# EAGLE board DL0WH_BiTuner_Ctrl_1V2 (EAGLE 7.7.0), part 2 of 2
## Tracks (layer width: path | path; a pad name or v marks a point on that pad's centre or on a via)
+3V3  (via drill 0.3)
  Top 0.152: R0913.2 10.48,30.48 13.02,33.02 | 19.21,26.83 18.72,27.32 R0971.1 15.24,27.94 v15.56,28.26 | 8.27,27.61 v8.26,27.62
  Top 0.254: U0601.3 28.18,45.95 27.94,45.72 | U0701.3 44.69,45.95 44.45,45.72 | U0801.3 61.2,45.95 60.96,45.72 | C0601.2 27.78,45.09 27.73,45.14 27.04,45.14 26.04,44.13 v26.04,42.55 | C0701.2 44.03,45.3 42.55,43.81 v42.55,42.55 | C0801.2 60.54,45.3 59.05,43.81 v59.05,42.55 | v13.97,16.51 13.64,16.84 U0961.5 17.62,21.74 17.62,23.34 16.67,24.29
  Top 0.305: C1311.1 28.26,37.47 27.62,37.47 v26.67,36.83 | L1311.1 L1311.3 v26.67,36.83 | U1301.5 13.29,41.23 v13.34,41.27 | 27.94,45.72 C0601.2 | 44.45,45.72 C0701.2 | 60.96,45.72 C0801.2 | X0222.1 71.28,30.96 71.44,30.8 R0511.2 R0512.2 | v71.44,19.68 68.26,19.68 v67.94,19.37 | v26.67,36.83 26.67,33.34 26.35,33.02 25.4,33.02 | 25.4,33.02 13.02,33.02 | 24.61,32.23 19.21,26.83 16.67,24.29 16.19,23.81 8.41,23.81 8.26,23.97 8.26,26.67 R0903.2 8.27,27.61 | L0941.2 24.56,32.23 v23.34,32.23 24.61,32.23 | 25.4,33.02 24.61,32.23
  Bottom 0.152: 75.56,4.13 75.56,6.02 | v67.94,19.37 67.94,19.1 SJ0401.1 | C0951.1 15.89,28.59 v15.56,28.26 14.63,27.33 U0951.5 | 22.28,34.12 C0941.1 | U0962.14 13.89,14.61 | 12.08,14.14 C0962.1 | U0962.8 13.98,10.79 15.08,10.79 15.24,10.95 15.24,12.7 | 15.24,12.7 15.24,14.45 15.06,14.62 U0962.14 | U0962.11 13.94,12.7 15.24,12.7 | U0962.14 13.97,14.69
  Bottom 0.254: U0921.8 7.9,27.98 v8.26,27.62 | 13.89,14.61 12.54,14.61 12.08,14.14 | 13.97,14.69 v13.97,16.51
  Bottom 0.305: v26.67,36.83 26.67,38.42 R1321.2 R1322.2 26.04,41.27 26.25,41.91 | v13.34,41.27 17.78,41.27 19.05,42.55 v26.04,42.55 26.25,42.33 26.25,41.91 | v59.05,42.55 59.05,41.91 58.74,41.59 58.42,41.59 | 26.25,41.91 26.35,41.81 26.35,41.59 42.55,41.59 | 75.56,4.13 75.88,3.81 79.38,3.81 X0201.1 | 75.56,6.02 R0231.2 74.92,7.29 74.93,9.21 74.93,19.37 74.61,19.68 73.66,19.68 | v71.44,19.68 73.66,19.68 | 58.42,41.59 58.42,31.11 58.58,30.96 X0222.1 73.5,30.96 73.66,30.8 73.66,19.68 | C0921.1 8.56,27.32 v8.26,27.62 | 42.55,41.59 58.42,41.59 | v42.55,42.55 42.55,41.59 | 22.28,34.12 U0941.5 U0941.4 v23.35,32.24 v23.34,32.23
+5V  (via drill 0.3)
  Top 0.152: U1101.16 43.88,11.43 C1101.1 | 11.75,47.62 L1211.1
  Top 0.254: U1301.1 16.24,40.37 v15.88,40.01 15.24,39.37 U1301.8
  Top 0.305: U1201.9 9.26,57.52 8.89,57.15 8.89,52.07 12.04,48.92 L1211.1 v13.34,47.62 | U1301.1 16.24,41.64 v17.14,42.55 | 11.75,47.62 3.81,47.62 1.27,44.45 1.27,14.29 8.26,7.3 | 8.26,7.3 14.29,1.27 47.62,1.27 47.94,1.59 47.94,7.94 46.35,9.53 46.35,11.12 C1101.1 | 8.26,7.3 35.24,34.29 78.74,34.29 82.55,30.48 | U1001.16 85.41,48.9 86.36,49.85 86.36,51.12 C1001.1 86.38,51.44 94.61,51.44 94.93,51.12 94.93,30.8 94.61,30.48 82.55,30.48 | 82.55,30.48 arc60 D1221.C
  Bottom 0.152: 14.82,35.14 15.24,35.56 15.24,39.37 v15.88,40.01
  Bottom 0.305: C1222.1 C1223.1 13,45.73 13.02,45.09 13.34,44.77 15.88,44.77 16.19,44.45 16.19,43.5 C1301.1 16.51,43.18 v17.14,42.55 | C1222.1 C1221.1 13.34,50.5 13.34,51.44 17.14,51.44 19.04,53.33 R1211.2 | C1222.1 13.32,47.64 v13.34,47.62 | R1302.2 14.82,35.14
+12V  (via drill 0.3)
  Top 0.254: U0601.6 30.12,46.08 30.48,45.72 | C0603.1 32.28,45.3 32.07,45.09 30.64,45.09 30.62,45.1 C0602.1 | U0701.6 46.63,46.08 46.99,45.72 | C0703.1 48.79,45.3 48.58,45.09 47.15,45.09 47.13,45.1 C0702.1 | U0801.6 63.15,46.08 63.5,45.72 | C0803.1 65.3,45.3 65.09,45.09 63.66,45.09 63.64,45.1 C0802.1
  Top 0.305: C0602.1 30.48,45.72 v31.43,45.72 | C0702.1 46.99,45.72 v47.94,45.72 | C0802.1 63.5,45.72 v64.45,45.72 | U1201.11 10.5,56.22 v10.16,55.88 | U1201.12 10.47,55.57 v10.16,55.88 | U1201.13 10.5,54.92 10.16,55.26 v10.16,55.88
  Bottom 0.305: 7.62,55.24 C1202.1 | C1204.1 v10.16,55.88 11.43,57.15 11.43,58.42 12.7,59.69 21.59,59.69 22.86,58.42 22.86,46.99 24.13,45.72 v31.43,45.72 v47.94,45.72 v64.45,45.72 70.48,45.72 78.74,53.98 78.74,64.77 | 78.74,64.77 X1602.17 X1602.18 X1602.20 X1602.19 78.74,64.77
  Bottom 0.406: C1204.1 C1203.1 C1202.1 C1201.1 5.73,55.88 X1211.1
-1V5  (via drill 0.3)
  Top 0.152: 36.45,37.88 L0943.1
  Top 0.254: U0961.2 12.7,21.91 13.03,22.24 C0952.1 12.7,22.72 v12.7,23.02
  Top 0.305: C0943.1 36.45,37.88 | v36.2,37.47 36.2,38.05 L0943.1 | v12.7,23.02 v16.67,23.02 | v33.34,30.48 v29.53,26.67
  Bottom 0.254: v12.7,23.02 U0951.2
  Bottom 0.305: C0945.2 R0945.2 33.34,30.97 v33.34,30.48 | C0945.2 32.07,33.5 | C0945.2 33.18,33.5 36.2,36.51 v36.2,37.47 | v29.53,26.67 20.32,26.67 v16.67,23.02
CAT_DTE_CTS
  Top 0.152: X1153.1 33.66,14.61 35.88,14.61 36.2,14.92 U1101.7
  Bottom 0.152: C1153.1 22.01,4.66 X1153.1
CAT_DTE_RTR
  Top 0.152: X1153.2 30.54,16.57 U1101.8
  Bottom 0.152: C1154.1 16.93,4.66 X1153.2
CAT_DTE_RXD
  Top 0.152: U1101.14 41.27,8.26 X1151.1
  Bottom 0.152: C1151.1 44.87,4.66 X1151.1
CAT_DTE_TXD
  Top 0.152: U1101.13 40.01,4.45 X1151.2
  Bottom 0.152: C1152.1 39.79,4.66 X1151.2
CAT_MX_C1N
  Top 0.152: C1102.2 46.04,14.61 41.59,14.61 41.27,14.92 U1101.3
CAT_MX_C1P
  Top 0.152: U1101.1 44.2,16.51 C1102.1
CAT_MX_C2M
  Top 0.152: U1101.5 38.73,18.41 40.01,19.69 C1103.2
CAT_MX_C2P
  Top 0.152: U1101.4 40.01,18.1 41.27,19.68 C1103.1
CAT_MX_VM
  Top 0.152: U1101.6 37.47,18.73 36.51,19.69 C1105.1
CAT_MX_VP
  Top 0.152: U1101.2 42.55,18.41 44.45,20.32 C1104.1
GND  (via drill 0.3)
  Top 0.152: U0601.7 U0601.8 31.43,47.94 v31.75,48.26 32.08,47.94 U0601.9 U0601.10 | U0701.7 U0701.8 47.94,47.94 v48.26,48.26 48.59,47.94 U0701.9 U0701.10 | U0801.7 U0801.8 64.44,47.94 v64.77,48.26 65.09,47.94 U0801.9 U0801.10 65.75,46.7 65.72,46.67 | 32.7,56.2 32.7,56.7 U0601.23 | 30.8,56.2 30.8,56.7 U0601.26 | U0601.25 31.43,56.2 | U0601.24 32.08,56.2 32.07,56.2 | U0801.26 63.8,56.22 63.82,56.2 | U0801.25 64.44,56.2 64.45,56.2 | U0801.24 65.09,56.2 | U0801.23 65.75,56.22 65.72,56.2 | S0212.1 | 57.78,17.94 57.61,18.1 C0311.2 | U0101.31 71.84,14.21 71.75,14.29 70.8,14.29 70.48,14.61 v70.48,16.51 66.99,16.51 v66.04,17.14 | U0101.63 65.34,23.25 v67.31,21.27 | R0441.1 59.05,16.67 | 53.02,3.87 H1721.B3,0 53.02,3.81 | 84.45,51.12 C1001.2 | 64.14,30.8 C0451.2 63.18,30.8 | 57.96,29.21 C0331.+ | C0803.2 65.83,43.6 66.04,43.81 | v14.61,28.26 13.97,27.62 D0971.C 14.42,26.67 17.46,26.67 v17.62,26.51 | v30,37.47 30,36.67 30.16,36.51 | U0961.3 11.73,20.32 | C0952.2 11.76,22.36
  Top 0.254: 14.61,43.18 15.24,42.55 U1301.3 15.24,40.64 14.74,39.82 U1301.7 14.74,36.06 | U1301.10 16.24,35.92 | U0701.10 49.23,46.65 50.16,45.72 50.16,44.45 49.53,43.81 49.11,43.81 C0703.2 | 32.49,43.6 C0603.2 32.6,43.81 33.02,43.81 33.66,44.45 33.66,45.72 32.73,46.65 U0601.10 | U0701.26 47.28,56.22 47.31,56.2 | U0701.23 49.23,56.22 49.21,56.2 | U0701.25 47.94,56.2 | U0701.24 48.59,56.2 48.58,56.2 | X1401.GND 89.88,22.89 v89.85,22.86 | 65.72,43.81 66.04,43.81 66.36,43.81 66.67,44.13 66.67,45.72 65.72,46.67 | 11.73,20.32 X1501.4 | 11.76,22.36 U0961.3
  Top 0.305: U1201.10 9.88,56.87 v9.72,56.77 | U1201.6 17.78,56.22 | 17.78,56.22 18.12,56.22 18.41,56.52 | 18.41,56.52 20.3,56.52 C1205.1 v20.32,57.78 v17.46,60.64 | U1201.7 18.06,56.87 18.41,56.52 | 18.41,56.52 17.78,56.22 | U1201.15 10.44,53.62 v10.16,53.34 | U1201.16 10.53,52.97 v10.16,53.34 | v13.34,43.18 14.61,43.18 v14.61,48.9 14.61,51.44 14.29,51.75 14.29,52.07 | 16.24,35.92 15.88,35.56 15.24,35.56 14.74,36.06 | v17.14,36.83 16.51,36.83 16.51,36.9 U1301.10 | C0601.1 28.1,43.66 28.16,43.6 28.79,43.6 v29.21,43.18 | C0603.2 32.23,43.81 30.96,43.81 30.94,43.8 C0602.2 30.32,43.66 30.27,43.6 29.63,43.6 v29.21,43.18 | v28.57,34.92 C1311.2 28.89,35.88 29.84,35.88 30.16,36.2 30.16,36.51 30.16,40.64 | C0701.1 44.45,43.66 44.51,43.6 45.3,43.6 v45.72,43.18 | v45.72,43.18 46.14,43.6 46.77,43.6 46.83,43.66 C0702.2 47.13,43.8 47.15,43.81 48.58,43.81 48.79,43.6 C0703.2 | C0803.2 65.3,43.6 65.09,43.81 63.66,43.81 63.64,43.8 C0802.2 63.34,43.66 63.28,43.6 62.65,43.6 v62.23,43.18 | C0801.1 61.12,43.66 61.17,43.6 61.81,43.6 v62.23,43.18 | U1201.PAD4 14.29,52.07 | 14.29,52.07 10.48,52.07 10.16,52.39 v10.16,53.34 | v29.21,43.18 29.21,40.96 29.53,40.64 30.16,40.64 | 30.16,40.64 38.89,40.64 | 38.89,40.64 45.72,40.64 | 45.72,40.64 61.91,40.64 62.23,40.96 | 62.23,40.96 v62.23,43.18 | 45.72,40.64 v45.72,43.18 | 30.8,56.2 31.43,56.2 31.75,56.2 | 31.75,56.2 32.07,56.2 32.7,56.2 | 31.75,56.2 U0601.33 | U0701.33 48.26,56.2 | 48.26,56.2 47.94,56.2 47.31,56.2 | 48.26,56.2 48.58,56.2 49.21,56.2 | 63.82,56.2 64.45,56.2 64.77,56.2 | 64.77,56.2 65.09,56.2 65.72,56.2 | v64.77,51.44 U0801.33 64.77,56.2 | S0212.1 65.72,5.08 65.41,5.4 C0213.2 65.34,7.86 65.34,13.27 U0101.18 65.34,16.44 v66.04,17.14 66.36,17.46 66.36,20.32 66.67,20.64 66.99,20.64 67.31,20.95 v67.31,21.27 67.94,21.91 v72.07,21.91 72.42,22.3 U0101.47
  Top 0.305: S0212.1 v68.9,4.45 | R0441.1 58.09,17.77 57.78,17.94 | 59.05,16.67 v59.21,16.67 | 53.02,3.87 49.21,7.62 49.21,11.11 48.9,11.43 v48.58,11.43 C1101.2 | U1101.15 42.55,8.26 v44.77,6.03 | C1105.2 34.61,20.32 34.61,21.27 35.24,21.91 46.04,21.91 46.35,21.59 46.35,21.27 C1104.2 v46.99,20.32 | X1052.1 90.81,47.62 U1001.15 83.82,47.62 83.03,47.94 83.03,50.01 83.66,50.48 84.45,51.12 | 62.23,40.96 62.55,40.64 74.93,40.64 74.93,40.95 C1005.2 74.93,52.39 75.25,52.7 82.55,52.7 82.87,52.39 82.87,51.12 | C1001.2 82.87,51.12 | 82.87,51.12 C1004.2 | 64.14,30.8 v64.77,30.16 65.09,29.84 65.09,27.46 65.34,27.21 U0101.63 | 63.18,30.8 61.59,29.21 60.96,29.21 | 60.96,29.21 57.96,29.21 | C0332.2 60.96,29.21 | v48.58,14.61 57.44,14.61 v58.42,14.27 | C0943.2 38.73,40.48 38.89,40.64
  Bottom 0.152: R1301.1 X1511.3 | C1223.2 C1222.2 | 59.52,15.48 C0412.2 | C0410.2 71.44,21.27 v72.07,21.91 | C0402.2 70.47,16.21 v70.48,16.51 | C0401.2 66.34,17.16 v66.04,17.14 | C0403.2 67.25,21.53 v67.31,21.27 | 59.28,16.6 v59.21,16.67 | R0221.1 v64.77,30.16 | 14.59,31.11 C0951.2 14.59,28.27 v14.61,28.26 | C1152.2 38.1,1.27 | C1151.2 43.18,1.27 | C1154.2 15.24,1.27 | C1153.2 20.32,1.27 | C1051.2 93.88,63.18 94.93,63.18 | C1052.2 94.93,58.42 | C1053.2 93.88,40.32 95.25,40.32 | C0054.2 95.25,35.56 | v17.14,36.83 17.14,34.61 17.62,34.13 C0941.2 | D0942.C v30,37.47 32.07,35.4 32.07,34.78 R0946.1 | U0941.2 28.26,33.18 28.57,33.5 v28.57,34.92 | v10.16,33.02 11.43,34.29 | C0962.2 10.79,13.96 10.79,13.18 | 10.79,13.18 12.7,13.18 12.85,13.32 U0962.12 U0962.13 13.96,13.97 13.97,13.97 | U0962.4 17.96,12.68 17.94,12.7 | 17.94,12.7 17.78,12.86 17.78,14.45 17.94,14.61 19.09,14.61 U0962.1 | 17.94,12.7 15.24,10 11.59,10 11.43,10.16 11.43,11.91 10.79,12.54 10.79,13.18
  Bottom 0.254: U0921.4 4.65,29.96 | C0962.2 9.51,15.24 X1501.3
  Bottom 0.305: C1212.2 20.3,57.8 v20.32,57.78 | v10.16,53.34 C1204.2 C1203.2 C1202.2 C1201.2 | C1301.2 v13.34,43.18 12.38,41.91 X1511.4 | X1211.2 9.72,60.96 | 9.72,60.96 v9.72,56.77 | X1211.2 H1751.B3,0 6.35,71.12 90.81,71.12 H1761.B3,0 94.93,66.99 94.93,63.18 94.93,58.42 94.93,53.66 92.71,51.44 X1052.1 X1052.2 95.25,41.91 95.25,40.32 95.25,35.56 95.25,30.48 91.44,26.67 89.22,26.67 C1403.1 89.2,25.4 C1403.1 | X1501.2 H1711.B3,0 6.35,1.27 15.24,1.27 20.32,1.27 26.99,1.27 X1152.2 X1152.1 36.83,1.27 38.1,1.27 43.18,1.27 50.55,1.27 H1721.B3,0 | X1501.2 X1501.3 X1501.4 11.76,23.19 11.76,23.81 | X1501.5 X1501.2 | X1501.5 3.81,21.91 4.23,22.33 C0901.2 R0901.1 | U0951.3 11.76,23.81 | C0921.2 10.16,24.77 11.11,23.81 11.76,23.81 | X1511.2 3.81,34.71 C0911.2 R0911.1 4.13,32.28 4.13,30.48 4.65,29.96 | X1511.5 X1511.4 | X1511.2 X1511.5 | X1511.4 X1511.3 11.43,34.29 v13.97,31.75 14.45,31.27 14.59,31.11 | C1222.2 C1221.2 v14.62,48.91 v14.61,48.9 | X1211.2 1.27,58.42 1.27,44.45 X1511.5 | 9.72,60.96 17.46,60.96 | 17.46,60.96 21.59,60.96 30.48,52.07 U0601.33 v31.75,48.26 | v17.46,60.64 17.46,60.96 | v48.26,48.26 U0701.33 | v64.77,48.26 v64.77,51.44 | H1731.B3,0 92.71,15.24 v90.17,17.78 90.17,22.54 v89.85,22.86 87,22.86 86.68,23.18 86.68,25.08 87,25.4 87.77,25.4 R1402.1 C1403.1 | v68.9,4.45 71.75,4.45 72.55,5.24 R0232.1 74.92,3.51 75.56,2.86 80.96,2.86 81.28,3.17 X0201.3 X0201.5 82.55,3.17 82.87,2.86 84.77,2.86 85.09,3.17 85.09,3.81 | 59.52,15.48 59.21,15.4 59.04,15.22 C0413.2 58.9,13.81 v58.42,14.27 | X0601.2 X0601.4 85.09,30.48 89.22,26.35 C1403.1 | C0412.2 59.37,15.56 59.37,16.51 59.28,16.6
  Bottom 0.305: v44.77,6.03 50.8,6.03 55.56,1.27 90.17,1.27 H1731.B3,0 | v48.58,11.43 v48.58,14.61 48.58,18.73 v46.99,20.32 | X1501.5 2.54,21.59 2.54,35.56 X1511.2 | 85.09,3.81 X0201.9 | 85.09,3.81 H1731.B3,0
  other vias: 31.75,52.07 48.26,52.07 55.88,20.32 68.58,58.42
  pour Top: 0.32,3.32 0.32,69.71 arc-88 3,72.71 93.2,72.71 arc-98 96.2,69.71 96.2,3.32 arc-88 93.2,0.32 3,0.32 arc-78
  pour Bottom: 0.32,3.32 0.32,69.71 arc-88 3,72.71 93.2,72.71 arc-98 96.2,69.71 96.2,3.32 arc-88 93.2,0.32 3,0.32 arc-78
LM2611_NFB
  Bottom 0.152: R0946.2 C0945.1 R0945.1 U0941.3
LM2611_SW  (via drill 0.3)
  Top 0.305: C0942.1 30.21,33.02 29.23,32.05 | 29.23,32.05 L0941.1 | v27.78,34.13 27.78,33.66 28.1,33.34 28.1,33.18 29.23,32.05
  Bottom 0.305: U0941.1 27.77,34.12 v27.78,34.13
LM53603_BIAS  (via drill 0.3)
  Top 0.152: U1201.5 18.74,55.57 19.05,55.88 v21.59,55.88
  Bottom 0.152: R1211.1 19.7,55.26 20.32,55.88 v21.59,55.88
  Bottom 0.305: R1211.1 C1212.1
LM53603_CBOOT
  Top 0.152: U1201.3 19.39,54.27 20,53.66 20.3,53.34
  Top 0.305: 20.3,53.34 C1211.2
LM53603_SW
  Top 0.152: 18.41,52.97 19.1,52.97 19.68,52.39 20.3,52.07
  Top 0.305: U1201.1 18.41,52.97 18.41,53.34 18.14,53.62 U1201.2 | 20.3,52.07 C1211.1
  Top 0.406: L1211.2 16.54,50.19 18.41,52.07 18.41,52.97
LM53603_VCC
  Top 0.152: U1201.4 19.36,54.92 19.68,55.24 20.3,55.24
  Top 0.305: 20.3,55.24 C1205.2
LM_DA  (via drill 0.3)
  Top 0.305: C0942.2 31.43,35.4 32.54,36.51 v32.54,37.47 L0943.2
  Bottom 0.305: v32.54,37.47 32.54,37.9 D0942.A
MCU_NRST  (via drill 0.3)
  Top 0.152: C0213.1 61.59,7.62 61.28,7.3 S0212.2 | C0213.1 64.14,9.51 64.14,4.13 64.45,3.81 71.12,3.81 74.45,7.14 84.14,7.14 85.09,6.19 X0201.10 | U0101.7 63.28,19.75 63.18,19.84 v64.29,19.84 | C0213.1 64.12,10.46 v64.14,12.06
  Bottom 0.152: v64.14,12.06 64.14,13.34 64.77,13.97 64.77,19.37 v64.29,19.84
MCU_VBAT
  Top 0.152: U0101.1 63.13,22.75 63.18,23.5 63.18,26.99 TP_VBAT.TP C0451.1
MCU_VDD  (via drill 0.3)
  Top 0.152: U0101.32 72.34,14.66 71.75,15.24 v71.75,16.51 | U0101.19 65.84,15.36 v66.36,15.88 | U0101.64 64.84,22.48 v66.04,21.27 | L0411.1 58.58,15.56 v57.78,15.56
  Bottom 0.152: C0402.1 71.77,16.21 v71.75,16.51 71.75,18.73 71.44,19.05 SJ0401.2 | C0403.1 65.95,21.5 v66.04,21.27 66.04,20.95 66.67,20.32 68.99,20.32 69.42,19.89 | SJ0401.2 69.42,19.89 | 69.42,19.89 69.85,20.32 69.85,21.21 C0410.1 | SJ0401.2 69.42,17.99 67.31,15.88 v66.36,15.88 66.34,15.86 C0401.1 66.04,12.86 64.14,10.95 60.48,10.95 57.15,13.97 57.15,15.08 v57.78,15.56
MCU_VDDA  (via drill 0.3)
  Top 0.152: U0101.13 61.73,16.8 L0411.2 60.54,14.55 v60.48,14.45
  Bottom 0.152: C0413.1 60.5,14.3 v60.48,14.45 60.9,14.99 C0412.1
MCU_VREF_M
  Top 0.152: U0101.12 61.08,17.3 R0441.2
MP_CAT_CTS_R  (via drill 0.3)
  Top 0.152: U1101.10 36.2,13.02 37.31,14.13 46.83,14.13 47.62,14.92 47.62,25.4 47.94,25.72 v55.56,25.72
  Bottom 0.152: v55.56,25.72 R1103.2
MP_CAT_RTR_R
  Top 0.152: U1101.9 R1104.2
MP_CAT_RXD_R
  Top 0.152: U1101.11 37.47,12.7 37.62,13.65 44.61,13.65 45.09,12.38 58.74,12.38 59.05,12.06 59.05,10.79 R1101.2
MP_CAT_TXD_R
  Top 0.152: U1101.12 R1102.2
MP_RS_CTS_R  (via drill 0.3)
  Top 0.152: R1003.2 v82.55,14.61 | v82.87,40.96 83.19,41.27 U1001.10
  Bottom 0.152: v82.55,14.61 82.55,28.89 82.23,29.21 76.83,29.21 75.88,30.16 75.88,31.43 82.87,38.42 v82.87,40.96
MP_RS_RTR_R
  Top 0.152: U1001.9 86.68,40.01 87,39.69 R1004.2
MP_RS_RXD_R  (via drill 0.3)
  Top 0.152: U1001.11 83.82,42.55 83.19,43.18 v82.87,43.18 | v60.96,33.02 56.83,33.02 56.52,32.7 v56.52,22.23
  Bottom 0.152: v82.87,43.18 81.28,43.18 79.06,40.96 79.06,38.42 73.66,33.02 v60.96,33.02 | v56.52,22.23 59.05,19.68 R1001.2
MP_RS_TXD_R
  Top 0.152: U1001.12 86.68,43.81 87,43.5 R1002.2
N$12
  Top 0.152: U0601.22 33.38,58.48 R0611.2
N$13
  Top 0.152: U0701.22 49.88,58.48 R0711.2
N$15
  Top 0.152: U0801.22 66.39,58.48 R0811.2
OPA_FB  (via drill 0.3)
  Top 0.152: v16.35,12.22 v17.94,10.64
  Bottom 0.152: R0963.1 15.88,12.7 v16.35,12.22 | v17.94,10.64 19.05,10.64 19.04,10.79 U0962.7
OPA_PULL  (via drill 0.3)
  Top 0.152: R0962.2 11.73,14.75 11.75,14.61 11.91,14.45 v11.91,12.54
  Bottom 0.152: U0962.9 11.96,11.38 11.91,11.43 v11.91,12.54
PA0
  Top 0.152: U0101.14 62,16.3 61.91,16.19 61.91,14.29 62.23,13.97 62.23,13.18 62.07,13.02 61.28,13.02 60.96,12.7 60.96,11.11 60.64,10.79 R1101.1
PA1  (via drill 0.3)
  Top 0.152: U0101.15 63.53,15.75 v63.98,15.24 | R1102.1 v38.73,6.35 | v61.44,13.65 v47.62,13.65
  Bottom 0.152: v63.98,15.24 62.39,13.65 v61.44,13.65 | v47.62,13.65 46.04,13.65 v38.73,6.35
PA3
  Top 0.152: U0101.17 64.83,13.59 64.77,13.26 63.59,13.26 63.5,13.18 63.5,12.64 62.87,12.06 R0922.1
PA5
  Top 0.152: U0101.21 66.84,12.54 66.36,11.75 R0621.1
PA6  (via drill 0.3)
  Top 0.152: U0101.22 67.34,12.73 v67.31,12.06
  Bottom 0.152: R0622.1 v67.31,12.06
PA7
  Top 0.152: U0101.23 67.84,12.81 R0623.1
PA9  (via drill 0.3)
  Top 0.152: U0101.42 81.85,19.8 v85.09,16.51 | v88.27,18.73 88.39,19.05
  Top 0.305: X1401.VBUS 89.64,20.29 88.39,19.05 PF1411.1
  Bottom 0.152: v85.09,16.51 87.95,16.51 88.27,16.83 v88.27,18.73
PA10
  Top 0.152: X1401.ID 92.69,22.24 93.03,21.91 93.03,18.73 91.12,16.83 87.31,16.83 86.68,17.46 86.68,20 86.36,20.3 U0101.43
PA11
  Top 0.152: X1401.D- 78.25,20.94 78.06,20.8 U0101.44
PA12
  Top 0.152: X1401.D+ 78.11,21.59 77.77,21.3 U0101.45
PA13  (via drill 0.3)
  Top 0.152: U0101.46 75.25,21.91 v75.88,21.91
  Bottom 0.152: 78.42,6.67 78.42,21.59 78.11,21.91 v75.88,21.91 | X0201.2 79.38,5.71 78.42,6.67 | R0231.1 78.42,6.67
PA14  (via drill 0.3)
  Top 0.152: U0101.49 72.36,24.1 73.34,24.13 v76.2,24.13 | v78.42,5.08 78.42,5.56 79.53,6.67 80.8,6.67 81.28,6.19 X0201.4
  Bottom 0.152: v78.42,5.08 76.37,5.08 R0232.2 | v76.2,24.13 79.38,24.13 79.63,23.88 79.63,7.84 81.28,6.19 X0201.4
PA15  (via drill 0.3)
  Top 0.152: U0101.50 71.91,24.02 v71.91,23.5
  Bottom 0.152: R1103.1 71.91,25.61 v71.91,23.5
PB0
  Top 0.152: U0101.26 69.34,11.87 69.53,11.43 R0624.1
PB1  (via drill 0.3)
  Top 0.152: U0101.27 69.84,12.53 v69.98,12.06
  Bottom 0.152: v69.98,12.06 R0724.1
PB2
  Top 0.152: U0101.28 70.34,12.53 71.12,11.75 R0824.1
PB6  (via drill 0.3)
  Top 0.152: X0601.1 76.83,27.3 72.72,27.3 R0512.1 72.71,27.62 72.39,27.94 68.74,27.94 v67.84,27.04 U0101.58 | v55.56,26.99 33.81,26.99 20.95,14.13 v20.64,14.13
  Bottom 0.152: v55.56,26.99 67.79,26.99 67.84,26.94 v67.84,27.04 | v20.64,14.13 20.48,13.97 U0962.2
PB7  (via drill 0.3)
  Top 0.152: U0101.59 67.33,23.5 67.47,23.34 v67.94,23.34 | v54.93,25.08 v48.58,25.08 | v46.67,25.08 42.23,25.08 v39.69,22.54 | R1104.1 v34.92,6.35
  Bottom 0.152: v67.94,23.34 67.94,24.92 67.79,25.08 v54.93,25.08 | v48.58,25.08 v46.67,25.08 | v34.92,6.35 34.92,17.78 v39.69,22.54
PB9  (via drill 0.3)
  Top 0.152: X0601.3 78.11,26.04 71.6,26.04 71.44,26.19 R0511.1 71.42,27.3 v69.85,27.3 | U0101.62 65.84,26.15 v66.04,26.35 | v54.93,26.35 34.13,26.35 v21.11,13.34
  Bottom 0.152: v69.85,27.3 68.9,26.35 v66.04,26.35 v54.93,26.35 | v21.11,13.34 19.12,13.34 U0962.3
PB10  (via drill 0.3)
  Top 0.152: U0101.29 70.84,12.66 72.39,11.11 v80.96,11.11 | v88.9,42.55 88.9,43.02 88.42,43.4 R1002.1
  Bottom 0.152: v80.96,11.11 80.96,24.45 80.64,24.77 76.83,24.77 74.61,26.99 74.61,32.7 80.33,38.42 80.33,40.96 81.6,42.23 88.58,42.23 v88.9,42.55
PB11
  Top 0.152: U0101.30 71.34,12.64 71.75,12.22 75.88,12.22 76.04,12.38 R0626.1 76.2,12.38
PB12
  Top 0.152: U0101.33 75.34,15.3 R1003.1
PB13  (via drill 0.3)
  Top 0.152: U0101.34 75.6,15.8 76.04,16.19 v81.6,16.19 | v88.9,40.64 88.9,40.11 R1004.1
  Bottom 0.152: v81.6,16.19 81.6,25.08 81.28,25.4 76.83,25.4 75.25,26.99 75.25,32.07 81.28,38.1 81.28,40.32 82.55,41.59 83.19,41.59 84.14,40.64 v88.9,40.64
PC0  (via drill 0.3)
  Top 0.152: U0101.8 63.62,19.25 64.77,19.25 v65.41,19.84 | v55.56,24.45 v49.21,24.45
  Bottom 0.152: v65.41,19.84 64.61,20.64 64.61,24.29 64.45,24.45 v55.56,24.45 | v49.21,24.45 46.04,24.45 45.4,25.08 36.83,25.08 30.8,31.11 18.1,31.11 17.14,30.16 17.14,28.26 15.56,26.67 15.56,25.4 15.89,25.07 R0972.2
PC1  (via drill 0.3)
  Top 0.152: U0101.9 62.83,18.73 62.07,18.73 v61.59,19.68
  Bottom 0.152: R1001.1 v61.59,19.68
PC2  (via drill 0.3)
  Top 0.152: D0971.A 15.04,26.22 R0971.2 v16.19,26.04 | U0101.10 63.35,18.25 62.71,18.26 61.91,18.26 60.8,19.37 60.8,20 v61.44,20.64 | v54.93,23.81 v48.58,23.81
  Bottom 0.152: v61.44,20.64 61.44,23.65 61.28,23.81 v54.93,23.81 | v48.58,23.81 43.81,23.81 43.18,24.45 36.2,24.45 30.16,30.48 18.41,30.48 18.1,30.16 18.1,27.94 v16.19,26.04
PC3
  Top 0.152: U0101.11 60.85,17.8 R0921.1
PC4  (via drill 0.3)
  Top 0.152: U0101.24 68.34,12.62 v68.58,12.06
  Bottom 0.152: R0625.1 v68.58,12.06
PC14_OSC32_IN
  Top 0.152: Q0321.2 57.8,23.81 | 57.8,23.81 C0331.- | 57.8,23.81 58.59,23.8 C0332.1 60.98,23.81 60.96,23.81 61.28,23.5 61.28,22.07 61.59,21.8 U0101.3
PC15_OSC32_OUT
  Top 0.152: U0101.4 60.8,21.3 60.49,21.57 Q0321.1 60.33,20 59.99,19.68 58.26,19.68 57.96,19.38 C0311.1
PH3_BOOT0
  Top 0.152: U0101.60 66.84,28.25 X0222.2
  Bottom 0.152: R0221.2 66.53,28.56 X0222.2
RELAY1
  Top 0.152: U0601.1 26.88,48.69 22.54,53.02 22.54,56.83 16.51,62.87 X1601.1
RELAY2
  Top 0.152: U0601.2 27.52,48.67 23.18,53.02 23.18,56.83 17.78,62.23 17.78,65.41 16.51,66.67 X1601.2
RELAY3
  Top 0.152: U0601.4 28.82,48.33 28.51,48.33 23.81,53.02 23.81,56.83 19.05,61.59 X1601.3
RELAY4
  Top 0.152: U0601.5 29.48,48.63 29.21,48.9 28.57,48.9 24.45,53.02 24.45,56.83 20.32,60.96 20.32,65.41 19.05,66.67 X1601.4
RELAY5  (via drill 0.3)
  Top 0.152: U0601.12 34.02,48.31 v35.88,50.16
  Bottom 0.152: X1601.5 21.59,64.14 35.24,50.48 v35.88,50.16
RELAY6  (via drill 0.3)
  Top 0.152: U0601.13 34.67,48.33 35.56,49.21 35.88,49.21 36.51,49.85 v36.51,50.8
  Bottom 0.152: X1601.6 22.86,66.04 22.86,64.14 36.2,50.8 v36.51,50.8
RELAY7  (via drill 0.3)
  Top 0.152: U0601.15 35.98,48.36 37.15,49.53 v37.15,50.16
  Bottom 0.152: X1601.7 24.13,63.82 37.15,51.12 v37.15,50.16
RELAY8  (via drill 0.3)
  Top 0.152: U0601.16 36.62,48.05 37.78,49.21 v37.78,50.8
  Bottom 0.152: X1601.8 25.4,66.04 25.4,63.82 37.78,51.44 v37.78,50.8
RELAY9  (via drill 0.3)
  Top 0.152: U0601.17 36.62,57.58 36.72,57.9 v36.83,57.78
  Bottom 0.152: X1601.9 26.67,63.5 33.02,57.15 36.2,57.15 v36.83,57.78
RELAY10  (via drill 0.3)
  Top 0.152: U0601.18 35.98,58.2 v36.2,58.42
  Bottom 0.152: X1601.10 27.94,66.04 27.94,62.87 33.34,57.47 35.24,57.47 v36.2,58.42
RELAY11  (via drill 0.3)
  Top 0.152: U0601.20 34.67,58.17 34.92,58.42 v35.24,58.42
  Bottom 0.152: X1601.11 29.21,62.23 33.34,58.1 34.92,58.1 v35.24,58.42
RELAY12  (via drill 0.3)
  Top 0.152: U0601.21 34.02,58.47 v34.61,59.05
  Bottom 0.152: X1601.12 30.48,66.04 30.48,61.59 32.7,59.37 34.29,59.37 v34.61,59.05
RELAY13
  Top 0.152: U0601.28 29.48,61.23 31.75,63.5 X1601.13
RELAY14
  Top 0.152: U0601.29 28.82,61.53 30.48,63.18 30.48,66.04 X1601.14
RELAY15
  Top 0.152: X1601.15 33.02,66.04 33.02,68.26 32.7,68.58 28.26,68.58 27.94,68.26 27.94,62.55 27.52,62.13 U0601.31
RELAY16
  Top 0.152: U0601.32 26.88,62.44 25.4,63.82 25.4,68.9 25.72,69.22 33.97,69.22 34.29,68.9 X1601.16
RELAY17
  Top 0.152: X1601.17 36.83,60.96 39.37,58.42 39.37,52.7 43.38,48.69 U0701.1
RELAY18
  Top 0.152: U0701.2 44.03,48.67 40.01,52.7 40.01,58.42 38.1,60.33 38.1,66.04 X1601.18
RELAY19
  Top 0.152: X1601.19 39.37,59.69 40.64,58.42 40.64,52.7 45.09,48.26 45.4,48.26 45.4,47.49 U0701.4
RELAY20
  Top 0.152: U0701.5 45.98,48.63 45.72,48.9 45.09,48.9 41.27,52.7 41.27,58.42 40.96,58.74 40.96,65.09 39.37,66.67 X1601.20
RELAY21
  Top 0.152: U0701.12 50.53,48.31 57.15,54.93 X1602.1
RELAY22
  Top 0.152: U0701.13 51.19,48.33 57.78,54.93 57.78,63.5 58.42,64.14 58.42,66.04 X1602.2
RELAY23
  Top 0.152: U0701.15 52.48,48.36 58.42,54.29 58.42,62.23 59.69,63.5 X1602.3
RELAY24
  Top 0.152: U0701.16 53.13,48.37 59.05,54.29 59.05,61.91 60.96,63.82 60.96,66.04 X1602.4
RELAY25  (via drill 0.3)
  Top 0.152: U0701.17 53.13,57.58 v53.34,57.78
  Bottom 0.152: X1602.5 60.96,66.04 60.96,68.26 60.64,68.58 53.66,68.58 53.34,68.26 v53.34,57.78
RELAY26  (via drill 0.3)
  Top 0.152: U0701.18 52.48,58.2 v52.7,58.42
  Bottom 0.152: X1602.6 62.23,68.9 61.91,69.22 53.02,69.22 52.7,68.9 v52.7,58.42
RELAY27  (via drill 0.3)
  Top 0.152: U0701.20 51.19,57.85 v51.75,58.42
  Bottom 0.152: X1602.7 63.5,66.04 63.5,69.53 63.18,69.85 52.07,69.85 51.75,69.53 v51.75,58.42
RELAY28  (via drill 0.3)
  Top 0.152: U0701.21 50.53,58.47 v51.12,59.05
  Bottom 0.152: X1602.8 64.77,70.17 64.45,70.48 51.44,70.48 51.12,70.17 v51.12,59.05
RELAY29
  Top 0.152: X1602.9 66.04,66.04 66.04,68.26 65.72,68.58 46.35,68.58 45.98,68.21 U0701.28
RELAY30
  Top 0.152: X1602.10 67.31,68.9 66.99,69.22 45.72,69.22 45.34,68.83 U0701.29
RELAY31
  Top 0.152: X1602.11 68.58,66.04 68.58,69.53 68.26,69.85 44.45,69.85 44.03,69.44 U0701.31
RELAY32
  Top 0.152: X1602.12 69.85,70.17 69.53,70.48 43.81,70.48 43.38,70.06 U0701.32
RELAY33  (via drill 0.3)
  Top 0.152: U0801.1 57.99,47.42 v57.78,47.62
  Bottom 0.152: v57.78,47.62 56.52,47.62 56.2,47.94 56.2,50.8 59.69,54.29 72.07,54.29 72.39,54.61 X1602.13
RELAY34  (via drill 0.3)
  Top 0.152: U0801.2 60.55,48.36 60.33,48.58 v58.42,48.58
  Bottom 0.152: v58.42,48.58 57.15,48.58 56.83,48.9 56.83,50.48 60.01,53.66 73.34,53.66 73.66,53.98 73.66,66.04 X1602.14
RELAY35  (via drill 0.3)
  Top 0.152: U0801.4 61.84,48.01 60.64,49.21 v57.78,49.21
  Bottom 0.152: v57.78,49.21 57.47,49.53 57.47,50.16 60.33,53.02 74.61,53.02 74.93,53.34 X1602.15
RELAY36  (via drill 0.3)
  Top 0.152: U0801.5 62.49,48.63 62.23,48.9 61.59,48.9 60.64,49.85 v58.42,49.85
  Bottom 0.152: v58.42,49.85 60.96,52.39 75.88,52.39 76.2,52.7 76.2,66.04 X1602.16
RM_FWD
  Bottom 0.305: X1501.1 L0901.2
RM_REV
  Bottom 0.152: L0911.2 X1511.1
RS_DTE_CTS
  Top 0.152: U1001.7 81.6,41.27 81.92,40.96 81.92,38.73 82.55,38.1 X1053.1
  Bottom 0.152: C1053.1 91.86,38.95 X1053.1
RS_DTE_RTR
  Top 0.152: U1001.8 80.01,39.95 80.01,38.1 85.09,33.02 X1053.2
  Bottom 0.152: C0054.1 91.86,33.87 X1053.2
RS_DTE_RXD  (via drill 0.3)
  Top 0.152: v88.27,46.35 U1001.14
  Bottom 0.152: v88.27,46.35 88.9,46.99 88.9,60.33 89.53,60.96 X1051.1 91.86,61.81 C1051.1
RS_DTE_TXD  (via drill 0.3)
  Top 0.152: v88.9,45.09 U1001.13
  Bottom 0.152: v88.9,45.09 90.17,46.35 90.17,55.24 90.81,55.88 X1051.2 91.86,56.73 C1052.1
RS_MX_C1N1
  Top 0.152: U1001.3 78.74,46.35 77.47,47.62 76.84,47.62 C1002.2
RS_MX_C1P
  Top 0.152: U1001.1 78.42,48.9 77.79,49.53 76.84,49.53 C1002.1
RS_MX_C2M1
  Top 0.152: U1001.5 78.11,43.81 77.79,43.5 76.84,43.5 C1003.2
RS_MX_C2P
  Top 0.152: U1001.4 78.11,45.09 77.79,45.4 76.84,45.4 C1003.1
RS_MX_VM
  Top 0.152: U1001.6 78.74,42.55 77.47,41.27 77.15,41.27 C1005.1
RS_MX_VP
  Top 0.152: U1001.2 81.28,47.62 81.6,47.94 81.6,49.53 81.28,49.85 80.01,49.85 79.69,50.16 79.69,51.12 C1004.1
SPI_DRV_!RST  (via drill 0.3)
  Top 0.152: U0701.27 46.63,61.88 v46.67,61.91 v54.61,61.91 | U0801.27 63.15,61.88 v63.18,61.91 72.71,61.91 73.03,61.59 v73.03,42.86 | U0601.27 30.12,59.65 v32.38,61.91 | v61.28,36.2 v51.75,36.2
  Bottom 0.152: v46.67,61.91 v32.38,61.91 | v54.61,61.91 v63.18,61.91 | v73.03,42.86 73.03,39.37 69.85,36.2 v61.28,36.2 | R0625.2 68.9,8.26 67.63,6.99 65.09,6.99 63.82,8.26 56.83,8.26 52.07,13.02 52.07,35.88 v51.75,36.2
SPI_DRV_C_!CS  (via drill 0.3)
  Top 0.152: v50.16,39.69 50.48,40.01 v62.23,40.01 | v60.33,41.59 53.98,41.59 51.84,43.73 U0701.14
  Bottom 0.152: R0724.2 70.48,7.62 68.58,5.71 64.45,5.71 63.18,6.99 56.2,6.99 50.8,12.38 50.8,35.24 50.16,35.88 v50.16,39.69 | v62.23,40.01 62.23,41.27 61.91,41.59 v60.33,41.59
SPI_DRV_EXT_!CS  (via drill 0.3)
  Top 0.152: R0824.2 v71.12,8.26 | U0801.14 68.34,45.95 70.17,44.13 v70.17,42.86 | v60.33,38.1 v49.21,38.1
  Bottom 0.152: v71.12,8.26 71.12,6.99 69.22,5.08 64.14,5.08 62.87,6.35 55.88,6.35 50.16,12.06 50.16,34.92 49.21,35.88 v49.21,38.1 | v70.17,42.86 70.17,39.37 68.9,38.1 v60.33,38.1
SPI_DRV_L_!CS  (via drill 0.3)
  Top 0.152: U0601.14 35.33,45.95 35.88,45.4 v35.88,43.81 | R0624.2 v69.53,8.26 | v61.28,38.73 v50.8,38.73
  Bottom 0.152: v35.88,43.81 44.13,43.81 45.09,44.77 51.44,44.77 52.39,43.81 60.64,43.81 61.59,44.77 66.67,44.77 69.53,42.23 69.53,39.69 68.58,38.73 v61.28,38.73 | v69.53,8.26 69.53,7.94 67.94,6.35 64.77,6.35 63.5,7.62 56.52,7.62 51.44,12.7 51.44,35.56 50.8,36.2 v50.8,38.73
SPI_DRV_PWM  (via drill 0.3)
  Top 0.152: v44.77,61.28 44.69,61.2 U0701.30 44.69,55.8 v42.86,53.98 | U0801.30 61.2,61.2 v61.28,61.28 | v47.94,61.28 v55.56,61.28 | U0601.30 28.18,55.33 v28.26,55.24 | v69.85,61.28 72.07,61.28 72.39,60.96 72.39,45.4 v72.07,45.09 | R0626.2 v83.5,12.38 | v77.47,38.1 v80.96,34.61 | v88.9,29.21 v83.5,23.81
  Bottom 0.152: v44.77,61.28 v47.94,61.28 | v55.56,61.28 v61.28,61.28 v69.85,61.28 | v42.86,53.98 38.1,49.21 35.56,49.21 29.53,55.24 v28.26,55.24 | v72.07,45.09 73.66,43.5 73.66,39.37 73.98,39.05 77.15,39.05 77.47,38.73 v77.47,38.1 | v83.5,12.38 v83.5,23.81 | v80.96,34.61 83.5,32.07 86.04,32.07 v88.9,29.21
SPI_DRV_SCLK  (via drill 0.3)
  Top 0.152: U0601.11 33.38,46.63 34.61,45.4 v34.61,43.18 | U0701.11 49.88,46.63 51.12,45.4 v51.12,43.18 | U0801.11 66.39,46.63 68.9,44.13 v68.9,41.91 | R0621.2 v66.36,8.89 | v54.61,39.37 v60.33,39.37
  Bottom 0.152: v34.61,43.18 44.45,43.18 45.4,44.13 50.16,44.13 v51.12,43.18 60.96,43.18 61.91,44.13 66.36,44.13 v68.9,41.91 68.9,40.01 68.26,39.37 v60.33,39.37 | v66.36,8.89 65.09,10.16 57.78,10.16 53.98,13.97 53.98,34.61 54.61,35.24 v54.61,39.37
SPI_DRV_SI  (via drill 0.3)
  Top 0.152: U0701.19 51.84,55.48 v52.39,54.93 | U0801.19 68.34,55.8 v68.9,55.24 70.8,53.34 v70.8,41.91 | U0601.19 35.33,55.48 v35.88,54.93 | R0623.2 v67.94,8.26 | v61.28,37.47 v52.7,37.47
  Bottom 0.152: v68.9,55.24 68.58,54.93 v52.39,54.93 v35.88,54.93 | v70.8,41.91 70.8,39.05 69.22,37.47 v61.28,37.47 | v67.94,8.26 67.31,7.62 65.41,7.62 64.14,8.89 57.15,8.89 52.7,13.34 v52.7,37.47
SPI_DRV_SO  (via drill 0.3)
  Top 0.152: v54.29,60.33 54.19,60.22 R0711.1 48.16,60.22 v47.94,60.33 | v65.09,60.33 65.94,59.91 R0811.1 71.22,60.02 71.44,59.69 v71.44,42.86 | R0611.1 35.46,60.22 v35.56,60.33 | v60.33,36.83 v53.66,36.83
  Bottom 0.152: v54.29,60.33 v65.09,60.33 | v35.56,60.33 v47.94,60.33 | v71.44,42.86 71.44,38.73 69.53,36.83 v60.33,36.83 | R0622.2 67.31,8.57 66.99,8.26 65.72,8.26 64.45,9.53 57.47,9.53 53.34,13.65 53.34,36.51 v53.66,36.83
SWR_IN_FWD  (via drill 0.3)
  Top 0.152: R0903.1 6.97,26.05 v7.3,25.72
  Bottom 0.152: R0902.2 7.62,25.4 v7.3,25.72 4.8,28.22 U0921.1
SWR_IN_FWD_HI
  Bottom 0.305: C0901.1 5.93,22.64 6.35,22.23 L0901.1 | C0901.1 R0901.2 | C0901.1 7.2,22.86 R0902.1
SWR_IN_REV  (via drill 0.3)
  Top 0.152: R0913.1 8.24,30.81 v7.3,31.75
  Bottom 0.152: R0912.2 7.62,32.07 v7.3,31.75 7.9,31.15 U0921.5
SWR_IN_REV_HI
  Bottom 0.152: C0911.1 5.73,34.62 6.35,35.24 L0911.1 | R0912.1 6.97,33.67 6.35,34.29 C0911.1 | R0911.2 C0911.1
SWR_OP1_OUT  (via drill 0.3)
  Top 0.152: D0951.C 12.7,25.08 13.02,24.77 v14.61,24.77
  Bottom 0.152: v14.61,24.77 14.58,24.74 U0951.1 13.64,22.7 R0961.1
SWR_OP2_IN  (via drill 0.3)
  Top 0.152: v11.75,18.73 v11.76,18.72 U0961.4 11.75,17.74 R0962.1 11.45,16.05 10.79,15.4 v10.79,11.59
  Bottom 0.152: C0963.1 11.76,19.53 R0961.2 v11.75,18.73 | U0962.6 17.73,11.38 15.88,9.53 10.95,9.53 10.79,9.68 v10.79,11.59
SWR_OP2_OUT  (via drill 0.3)
  Top 0.152: U0961.1 14.26,20.34 v14.29,20.32
  Bottom 0.152: R0963.2 15.4,18.75 C0963.2 | R0972.1 15.4,20.3 C0963.2 | v14.29,20.32 14.62,19.99 C0963.2
SWR_SEL_FWD  (via drill 0.3)
  Top 0.152: R0921.2 59.05,18.59 58.74,18.73 50.16,18.73 v48.58,20.32 | v9.21,28.57 12.06,28.57 12.38,28.89 18.73,28.89 v19.05,28.57
  Bottom 0.152: v48.58,20.32 47.62,21.27 43.18,21.27 41.27,23.18 34.92,23.18 29.53,28.57 v19.05,28.57 | U0921.7 8.82,28.96 v9.21,28.57
SWR_SEL_PWR  (via drill 0.3)  (1 unrouted)
  Top 0.152: D0951.A v12.7,27.94
  Bottom 0.152: 11.16,29.46 U0921.6 6.6,29.46 6.1,28.96 U0921.2 | 11.43,29.2 11.43,28.57 11.76,28.25 U0951.4 12.09,27.33 v12.7,27.94
SWR_SEL_REV  (via drill 0.3)
  Top 0.152: R0922.2 60.31,12.08 59.37,13.02 v49.45,13.02 | v6.03,30.16 6.67,29.53 v20,29.53
  Bottom 0.152: v49.45,13.02 49.45,20.4 47.62,22.23 43.81,22.23 42.23,23.81 35.56,23.81 29.84,29.53 v20,29.53 | U0921.3 5.08,29.53 5.4,29.53 v6.03,30.16
TPS_LBI  (via drill 0.3)
  Top 0.152: U1301.6 14.24,36.47 13.97,36.2 v13.32,36.2
  Bottom 0.152: R1302.1 v13.32,36.2 | 13.12,36.62 13.12,36.41
  Bottom 0.305: 13.12,36.62 R1301.2 | 13.12,36.41 v13.32,36.2
TPS_LBO  (via drill 0.3)
  Top 0.152: 15.74,42.41 17.14,43.81 23.5,43.81 24.77,42.55 v24.77,41.27
  Top 0.305: U1301.2 15.74,42.41
  Bottom 0.305: R1322.1 24.55,41.06 v24.77,41.27
TPS_PG  (via drill 0.3)
  Top 0.152: U1301.4 14.74,40.77 v13.65,39.69
  Bottom 0.152: R1321.1 24.55,39.27 v24.13,39.37 18.73,39.37 17.78,40.64 14.61,40.64 v13.65,39.69
TPS_SW
  Top 0.254: U1301.9 15.74,38.6 15.88,38.73
  Top 0.305: 15.88,38.73 17.24,38.73 18.73,36.83 L1311.4 L1311.2
USB_SHIELD
  Bottom 0.305: X1401.JSHIELD 93.36,19.09 X1401.JSHIELD@3 X1401.JSHIELD@4 X1401.JSHIELD@5 X1401.JSHIELD@6 93.36,24.11 X1401.JSHIELD@2 91.63,24.11 C1403.2 R1402.2
VDDUSB  (via drill 0.3)
  Top 0.152: U0101.48 81.6,22.8 | 84.88,22.8 v85.09,22.54 | v85.09,18.73 85.09,18.92 PF1411.2
  Top 0.305: 84.88,22.8 81.6,22.8 81.6,25.4 83.71,27.51 D1221.A
  Bottom 0.305: v85.09,22.54 v85.09,18.73

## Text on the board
tPlace: 2 | 22 | 36 | 12V | 12V | DL0WH BiTuner Ctrl V1.2 / (C) 2019 | 23 | - | 1 | 21 | 22 | 35 | 12V | 12V | BAT | OUTPUT A | OUTPUT B | RXD | RS232 | TXD | 12V | + | GND | FWD | GND | CTS | BOOT0 | I2C | RTR | SCL | SDA | USB | REV | CAT Ifc. | SWD | RTR | CTS | GND | GND | TXD | RXD | RESET
Measures: 4x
